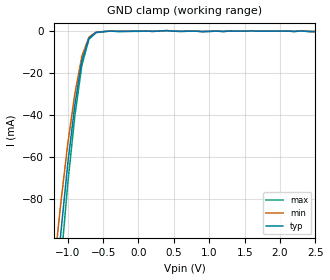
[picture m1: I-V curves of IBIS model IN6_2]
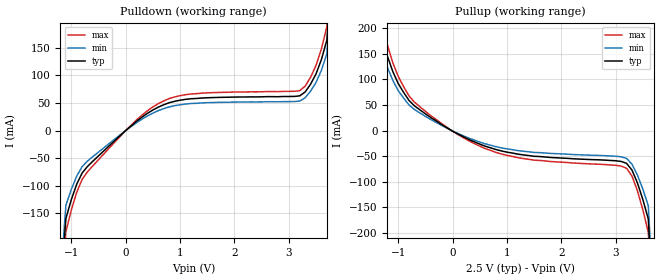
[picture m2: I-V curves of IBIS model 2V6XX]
[IBIS Ver]   2.1
[File name]   524_2.ibs
[File Rev]   2.0
[Date]   9/13/06
[Source]   ICS MicroClock Applications Engineering 2
[Disclaimer] This information is for modeling purposes only, and is
(C) Copyright Integrated Circuit Systems, Inc. 1997-2001
   All rights reserved
ICS hereby grants the user of this IBIS model a non-exclusive,
nontransferable license to use this IBIS model under the following terms.
Before using this IBIS model, the user should read this license.
If the user does not accept these terms,  the IBIS model should be
returned to ICS within 30 days.
   The user is granted this license only to use the IBIS model and
is not granted rights to sell, load, rent, lease or license the IBIS
model in whole or in part, or in modified form to anyone other than
user. User may modify the IBIS model to suit its specific
applications but rights to derivative works and such modifications
shall belong to ICS.
   This IBIS model is provided on an "AS IS" basis and ICS makes
absolutely no warranty with respect to the information contained
herein. ICS DISCLAIMS AND CUSTOMER WAIVES ALL WARRANTIES, EXPRESS
OR IMPLIED, INCLUDING WARRANTIES OF MERCHANTABILITY OR FITNESS FOR
A PARTICULAR PURPOSE. The entire risk as to quality and performance
is with the Customer. ACCORDINGLY, IN NO EVENT SHALL THE COMPANY BE
LIABLE FOR ANY DAMAGES, WHETHER IN CONTRACT OR TORT,INCLUDING ANY
LOST PROFITS OR OTHER INCIDENTAL, CONSEQUENTIAL, EXEMPLARY, OR
PUNITIVE DAMAGES ARISING OUT OF THE USE OR APPLICATION OF THE IBIS
model provided in this package. Further, ICS reserves the right to
make changes without notice to any product herein to improve
reliability, function, or design. ICS does not convey any license
under patent rights or any other intellectual property rights,
including those of third parties.
   ICS is not obligated to provide maintenance or support
for the licensed IBIS model.
[Component]   ICS524
[Manufacturer] Integrated Circuit Systems Inc.
[Package]
|   typ   min   max
R_pkg   40m   35m   45m
L_pkg   1.65nH   1.35nH   1.95nH
C_pkg   0.24pF   0.14pF   0.34pF
[pin]   signal_name   model_name   R_pin   L_pin   C_pin
   1   ICLK   IN6_2   58.6m   1.968nH   0.286pF
   2   Q0   2V6XX   55.5m   1.570nH   0.252pF
   3   Q1   2V6XX   55.5m   1.570nH   0.252pF
   4   NC   NC
   5   VDD   POWER
   6   Q2   2V6XX   55.5m   1.570nH   0.252pF
   7   Q3   2V6XX   55.5m   1.570nH   0.252pF
   8   GND   GND
| Models and submodels in the file (2): IN6_2 (Input), 2V6XX (Output)
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|   2.5V  INPUT  Model
| This model is suitable for ALL INPUT Pin
[Model]   IN6_2
Model_type   Input
Polarity   Non-Inverting
Vinl = 0.75V   | input logic "low" DC voltage
Vinh = 1.75V   | input logic "high" DC voltage
|   typ   min   max
C_comp   5pF   4pF   6pF
|   typ   min   max
[Voltage range]  2.5V   2.375V   2.625V
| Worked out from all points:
|   GND clamp passes 1 mA (typ) near -0.61 V on its own axis
[GND_clamp]
|Voltage I (typ)   I (min)   I (max)
-2.5V     -3A        -3A        -3A
-1.2V     -135.8mA   -115.4mA   -156.1mA
-1.1V     -97.7mA    -83.05mA   -112.4mA
-1V       -63.72mA   -54.16mA   -73.28mA
-900mV    -35.55mA   -30.22mA   -40.89mA
-800mV    -14.29mA   -12.15mA   -16.44mA
-700mV    -3.48mA    -2.958mA   -4.002mA
-600mV    -708uA     -601.8uA   -814.2uA
-400mV    -72.3uA    -61.47uA   -83.16uA
400mV     155uA      131.8uA    178.2uA
900mV     -299uA     -254.2uA   -343.8uA
2.5V      -299uA     -254.2uA   -343.8uA
|   ICS524 2.5V Clock Drive Model
| This model is suitable for all output pins on the
|  ICS524
[Model]   2V6XX
Model_type   Output
Polarity   Non-Inverting
Vmeas = 1.25V
Vref =  1.25V
Rref = 50.00000
Cref =  15pF
|   typ   min   max
C_comp   5pF   4pF   6pF
|   typ   min   max
[Voltage range]  2.5V   2.375V   2.625V
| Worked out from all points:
|   slope of the pulldown table from 0 to 0.375 V, typ, clamps not added: 12.7 ohm
|   slope of the pullup table from 0 to 0.375 V, typ, clamps not added: 19 ohm
[pulldown]
|Voltage I (typ)   I (min)   I (max)
-2.5V     -2A        -2A        -2A
-1.1V     -159.5mA   -135.5mA   -183.4mA
-900mV    -97.04mA   -82.48mA   -111.6mA
-700mV    -64.77mA   -55.06mA   -74.49mA
200mV     16.79mA    14.27mA    19.3mA
600mV     42.42mA    36.05mA    48.78mA
1.2V      57.54mA    48.91mA    66.18mA
3.2V      62.77mA    53.35mA    72.19mA
3.3V      69.81mA    59.34mA    80.28mA
3.5V      102.5mA    87.11mA    117.9mA
3.7V      163.8mA    139.2mA    188.4mA
5V        2A         2A         2A
[pullup]
|Voltage I (typ)   I (min)   I (max)
-2.5V     2A         2A         2A
-1.3V     184.4mA    156.7mA    212.1mA
-1.1V     115.6mA    98.28mA    133mA
-800mV    58.73mA    49.92mA    67.54mA
-400mV    25.33mA    21.53mA    29.13mA
200mV     -12.3mA    -10.45mA   -14.14mA
1.2V      -46.19mA   -39.26mA   -53.12mA
3.2V      -64.23mA   -54.59mA   -73.86mA
3.3V      -77.54mA   -65.91mA   -89.17mA
3.4V      -102.6mA   -87.23mA   -118mA
3.6V      -173.6mA   -147.5mA   -199.6mA
5V        -3A        -3A        -3A
[Ramp]
|   typ   min   max
dV/dt_r   1.10/0.58n   1.05/0.64n   1.55/0.52n
dV/dt_f   1.21/0.55n   1.15/0.60n   1.27/0.50n
